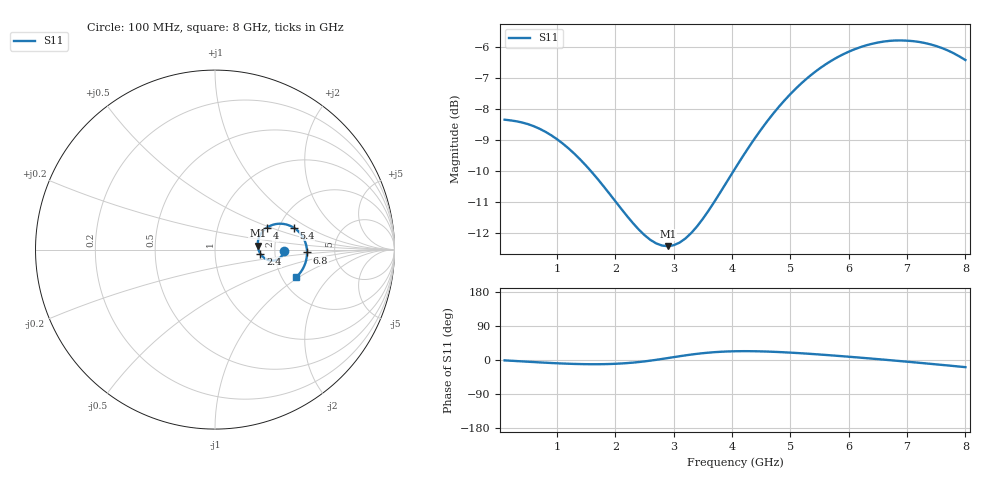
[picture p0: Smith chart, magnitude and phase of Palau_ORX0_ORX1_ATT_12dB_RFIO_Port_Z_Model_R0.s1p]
! Created Fri Jul 10 10:53:55 2020
! Palau ORX0/ORX1 RFIO Port Impedance Model.
! Attenuation : 12 dB.
! Revision		: R0.
! Impedance Mode 	: Balanced Differential-Mode.
! Impedance Format 	: Series Equivalent Differential Impedance (SEDZ).
# hz S ma R 50
! 1 Port Network Data from SP1.SP block
! freq  magS11  angS11
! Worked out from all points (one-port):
!   80 points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, 100 MHz to 8 GHz, reference 50 ohm
!   lowest |S11| = -12.4 dB at 2.9 GHz (marker M1), VSWR 1.63, Z = 81.2 + j3.7 ohm
!   |S11| at or under -10 dB: 1.577 GHz to 4.026 GHz (2.448 GHz wide, 87.4 % of centre)
!   S11 on the Smith chart (normalised r, x): 100 MHz: 2.24, -0.03; 2.4 GHz: 1.68, -0.09; 4 GHz: 1.73, +0.47; 5.4 GHz: 2.40, +0.74; 6.8 GHz: 3.10, -0.13; 8 GHz: 2.38, -0.95
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1e8  0.3826 -1.0
6e8  0.3734 -5.4
1.1e9  0.3499 -9.3
1.4e9  0.3297 -10.7
1.6e9  0.3145 -11.1
1.8e9  0.2985 -10.9
2.1e9  0.2748 -9.2
2.4e9  0.2544 -5.4
2.7e9  0.2416 0.5
2.9e9  0.2392 5.2
3.1e9  0.2424 9.9
3.3e9  0.2512 14.4
3.5e9  0.2649 18.0
4e9  0.3134 22.9
4.1e9  0.3245 23.2
4.4e9  0.3581 23.1
4.6e9  0.3801 22.2
4.8e9  0.4011 21.0
5.1e9  0.43 18.5
5.4e9  0.4552 15.6
5.7e9  0.476 12.2
6.1e9  0.4969 7.4
6.5e9  0.5094 2.3
6.8e9  0.5133 -1.8
7.1e9  0.5121 -5.9
7.3e9  0.5086 -8.7
7.6e9  0.4991 -13.0
8e9  0.4774 -18.9
